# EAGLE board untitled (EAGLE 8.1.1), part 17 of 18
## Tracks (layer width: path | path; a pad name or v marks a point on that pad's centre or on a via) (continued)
S$17259 (continued)
  Bottom 0: 77.97,164.06 77.65,164.08
S$17260
  Bottom 0: 77.65,164.08 77.39,164.03
S$17261
  Bottom 0: 77.39,164.03 75.39,166.04
S$17262
  Bottom 0: 75.39,166.04 75.32,166.1
S$17263
  Bottom 0: 75.32,166.1 75.25,166.15
S$17264
  Bottom 0: 75.25,166.15 75.16,166.18
S$17265
  Bottom 0: 75.16,166.18 75.08,166.2
S$17266
  Bottom 0: 75.08,166.2 74.99,166.21
S$17267
  Bottom 0: 74.99,166.21 68.93,166.21
S$17268
  Bottom 0: 68.93,166.21 68.75,166.33
S$17269
  Bottom 0: 68.75,166.33 68.45,166.44
S$17270
  Bottom 0: 68.45,166.44 68.12,166.46
S$17271
  Bottom 0: 68.12,166.46 67.8,166.4
S$17272
  Bottom 0: 67.8,166.4 67.79,166.38
S$17273
  Bottom 0: 67.79,166.38 80.91,179.51
S$17274
  Bottom 0: 80.91,179.51 81.03,179.51
S$17275
  Bottom 0: 81.03,179.51 81.03,177.8
S$17276
  Bottom 0: 81.03,177.8 81.04,177.72
S$17277
  Bottom 0: 81.04,177.72 81.08,177.65
S$17278
  Bottom 0: 81.08,177.65 81.14,177.6
S$17279
  Bottom 0: 81.14,177.6 81.21,177.56
S$17280
  Bottom 0: 81.21,177.56 81.28,177.55
S$17281
  Bottom 0: 81.28,177.55 81.67,177.55
S$17282
  Bottom 0: 81.67,177.55 79.01,174.88
S$17283
  Bottom 0: 79.01,174.88 78.97,174.83
S$17284
  Bottom 0: 78.97,174.83 78.93,174.77
S$17285
  Bottom 0: 78.93,174.77 78.9,174.71
S$17286
  Bottom 0: 78.9,174.71 78.89,174.64
S$17287
  Bottom 0: 78.89,174.64 78.88,174.57
S$17288
  Bottom 0: 78.88,174.57 78.88,166.19
S$17289
  Bottom 0: 78.88,166.19 78.71,166.03
S$17290
  Bottom 0: 78.71,166.03 78.54,165.75
S$17291
  Bottom 0: 78.54,165.75 78.46,165.43
S$17292
  Bottom 0: 78.46,165.43 78.46,165.11
S$17293
  Bottom 0: 78.46,165.11 78.54,164.79
S$17294
  Bottom 0: 78.54,164.79 78.71,164.52
S$17295
  Bottom 0: 78.71,164.52 78.95,164.3
S$17296
  Bottom 0: 78.95,164.3 79.24,164.15
S$17297
  Bottom 0: 79.24,164.15 79.56,164.08
S$17298
  Bottom 0: 79.56,164.08 79.88,164.1
S$17299
  Bottom 0: 79.88,164.1 80.19,164.21
S$17300
  Bottom 0: 80.19,164.21 80.45,164.4
S$17301
  Bottom 0: 80.45,164.4 80.66,164.65
S$17302
  Bottom 0: 80.66,164.65 80.78,164.95
S$17303
  Bottom 0: 80.78,164.95 80.83,165.27
S$17304
  Bottom 0: 80.83,165.27 80.78,165.59
S$17305
  Bottom 0: 80.78,165.59 80.66,165.89
S$17306
  Bottom 0: 80.66,165.89 80.45,166.15
S$17307
  Bottom 0: 80.45,166.15 80.19,166.33
S$17308
  Bottom 0: 80.19,166.33 79.88,166.44
S$17309
  Bottom 0: 79.88,166.44 79.76,166.44
S$17310
  Bottom 0: 79.76,166.44 79.76,167.73
S$17311
  Bottom 0: 79.76,167.73 79.78,167.71
S$17312
  Bottom 0: 79.78,167.71 80.02,167.45
S$17313
  Bottom 0: 80.02,167.45 80.31,167.26
S$17314
  Bottom 0: 80.31,167.26 80.64,167.16
S$17315
  Bottom 0: 80.64,167.16 80.99,167.14
S$17316
  Bottom 0: 80.99,167.14 81.34,167.2
S$17317
  Bottom 0: 81.34,167.2 81.65,167.35
S$17318
  Bottom 0: 81.65,167.35 81.92,167.57
S$17319
  Bottom 0: 81.92,167.57 82.13,167.86
S$17320
  Bottom 0: 82.13,167.86 82.25,168.18
S$17321
  Bottom 0: 82.25,168.18 82.3,168.53
S$17322
  Bottom 0: 82.3,168.53 82.25,168.87
S$17323
  Bottom 0: 82.25,168.87 82.13,169.2
S$17324
  Bottom 0: 82.13,169.2 81.92,169.48
S$17325
  Bottom 0: 81.92,169.48 81.65,169.71
S$17326
  Bottom 0: 81.65,169.71 81.34,169.86
S$17327
  Bottom 0: 81.34,169.86 80.99,169.92
S$17328
  Bottom 0: 80.99,169.92 80.64,169.9
S$17329
  Bottom 0: 80.64,169.9 80.31,169.79
S$17330
  Bottom 0: 80.31,169.79 80.02,169.61
S$17331
  Bottom 0: 80.02,169.61 79.78,169.35
S$17332
  Bottom 0: 79.78,169.35 79.76,169.34
S$17333
  Bottom 0: 79.76,169.34 79.76,174.38
S$17334
  Bottom 0: 79.76,174.38 82.49,177.1
S$17335
  Bottom 0: 82.49,177.1 82.53,177.17
S$17336
  Bottom 0: 82.53,177.17 82.56,177.2
S$17337
  Bottom 0: 82.56,177.2 82.56,177.24
S$17338
  Bottom 0: 82.56,177.24 82.6,177.3
S$17339
  Bottom 0: 82.6,177.3 82.6,177.36
S$17340
  Bottom 0: 82.6,177.36 82.62,177.42
S$17341
  Bottom 0: 82.62,177.42 82.62,177.55
S$17342
  Bottom 0: 82.62,177.55 83.06,177.55
S$17343
  Bottom 0: 83.06,177.55 83.14,177.56
S$17344
  Bottom 0: 83.14,177.56 83.21,177.6
S$17345
  Bottom 0: 83.21,177.6 83.27,177.65
S$17346
  Bottom 0: 83.27,177.65 83.31,177.72
S$17347
  Bottom 0: 83.31,177.72 83.32,177.8
S$17348
  Bottom 0: 83.32,177.8 83.32,179.51
S$17349
  Bottom 0: 83.32,179.51 83.92,179.51
S$17350
  Bottom 0: 83.92,179.51 83.75,179.31
S$17351
  Bottom 0: 83.75,179.31 83.62,179.01
S$17352
  Bottom 0: 83.62,179.01 83.57,178.69
S$17353
  Bottom 0: 83.57,178.69 83.62,178.37
S$17354
  Bottom 0: 83.62,178.37 83.75,178.07
S$17355
  Bottom 0: 83.75,178.07 83.97,177.82
S$17356
  Bottom 0: 83.97,177.82 84.24,177.65
S$17357
  Bottom 0: 84.24,177.65 84.55,177.56
S$17358
  Bottom 0: 84.55,177.56 84.88,177.56
S$17359
  Bottom 0: 84.88,177.56 85.19,177.65
S$17360
  Bottom 0: 85.19,177.65 85.46,177.82
S$17361
  Bottom 0: 85.46,177.82 85.67,178.07
S$17362
  Bottom 0: 85.67,178.07 85.81,178.37
S$17363
  Bottom 0: 85.81,178.37 85.86,178.69
S$17364
  Bottom 0: 85.86,178.69 85.81,179.01
S$17365
  Bottom 0: 85.81,179.01 85.67,179.31
S$17366
  Bottom 0: 85.67,179.31 85.5,179.51
S$17367
  Bottom 0: 85.5,179.51 100.08,179.51
S$17368
  Bottom 0: 100.08,179.51 100.08,177.8
S$17369
  Bottom 0: 100.08,177.8 100.09,177.72
S$17370
  Bottom 0: 100.09,177.72 100.13,177.65
S$17371
  Bottom 0: 100.13,177.65 100.18,177.6
S$17372
  Bottom 0: 100.18,177.6 100.25,177.56
S$17373
  Bottom 0: 100.25,177.56 100.33,177.55
S$17374
  Bottom 0: 100.33,177.55 100.72,177.55
S$17375
  Bottom 0: 100.72,177.55 97.88,174.71
S$17376
  Bottom 0: 97.88,174.71 97.83,174.66
S$17377
  Bottom 0: 97.83,174.66 97.8,174.6
S$17378
  Bottom 0: 97.8,174.6 97.77,174.53
S$17379
  Bottom 0: 97.77,174.53 97.75,174.47
S$17380
  Bottom 0: 97.75,174.47 97.75,174.4
S$17381
  Bottom 0: 97.75,174.4 97.75,165.99
S$17382
  Bottom 0: 97.75,165.99 97.59,165.75
S$17383
  Bottom 0: 97.59,165.75 97.51,165.43
S$17384
  Bottom 0: 97.51,165.43 97.51,165.1
S$17385
  Bottom 0: 97.51,165.1 97.59,164.79
S$17386
  Bottom 0: 97.59,164.79 97.67,164.67
S$17387
  Bottom 0: 97.67,164.67 95.44,166.9
S$17388
  Bottom 0: 95.44,166.9 95.38,166.94
S$17389
  Bottom 0: 95.38,166.94 95.32,166.98
S$17390
  Bottom 0: 95.32,166.98 95.26,167
S$17391
  Bottom 0: 95.26,167 95.19,167.02
S$17392
  Bottom 0: 95.19,167.02 95.12,167.03
S$17393
  Bottom 0: 95.12,167.03 91.92,167.03
S$17394
  Bottom 0: 91.92,167.03 88.5,170.45
S$17395
  Bottom 0: 88.5,170.45 88.61,170.72
S$17396
  Bottom 0: 88.61,170.72 88.65,171.07
S$17397
  Bottom 0: 88.65,171.07 88.61,171.41
S$17398
  Bottom 0: 88.61,171.41 88.48,171.74
S$17399
  Bottom 0: 88.48,171.74 88.27,172.02
S$17400
  Bottom 0: 88.27,172.02 88,172.25
S$17401
  Bottom 0: 88,172.25 87.69,172.4
S$17402
  Bottom 0: 87.69,172.4 87.34,172.46
S$17403
  Bottom 0: 87.34,172.46 86.99,172.44
S$17404
  Bottom 0: 86.99,172.44 86.66,172.33
S$17405
  Bottom 0: 86.66,172.33 86.36,172.15
S$17406
  Bottom 0: 86.36,172.15 86.13,171.89
S$17407
  Bottom 0: 86.13,171.89 85.95,171.58
S$17408
  Bottom 0: 85.95,171.58 85.86,171.24
S$17409
  Bottom 0: 85.86,171.24 85.86,170.9
S$17410
  Bottom 0: 85.86,170.9 85.95,170.56
S$17411
  Bottom 0: 85.95,170.56 86.13,170.25
S$17412
  Bottom 0: 86.13,170.25 86.36,169.99
S$17413
  Bottom 0: 86.36,169.99 86.66,169.8
S$17414
  Bottom 0: 86.66,169.8 86.99,169.7
S$17415
  Bottom 0: 86.99,169.7 87.34,169.68
S$17416
  Bottom 0: 87.34,169.68 87.69,169.74
S$17417
  Bottom 0: 87.69,169.74 87.87,169.83
S$17418
  Bottom 0: 87.87,169.83 91.42,166.27
S$17419
  Bottom 0: 91.42,166.27 91.48,166.23
S$17420
  Bottom 0: 91.48,166.23 91.53,166.19
S$17421
  Bottom 0: 91.53,166.19 91.6,166.16
S$17422
  Bottom 0: 91.6,166.16 91.66,166.15
S$17423
  Bottom 0: 91.66,166.15 91.73,166.14
S$17424
  Bottom 0: 91.73,166.14 94.94,166.14
S$17425
  Bottom 0: 94.94,166.14 97.01,164.06
S$17426
  Bottom 0: 97.01,164.06 96.7,164.08
S$17427
  Bottom 0: 96.7,164.08 96.45,164.03
S$17428
  Bottom 0: 96.45,164.03 94.81,165.67
S$17429
  Bottom 0: 94.81,165.67 94.74,165.74
S$17430
  Bottom 0: 94.74,165.74 94.67,165.78
S$17431
  Bottom 0: 94.67,165.78 94.58,165.81
S$17432
  Bottom 0: 94.58,165.81 94.5,165.84
S$17433
  Bottom 0: 94.5,165.84 94.4,165.84
S$17434
  Bottom 0: 94.4,165.84 88.3,165.84
S$17435
  Bottom 0: 88.3,165.84 88.28,165.89
S$17436
  Bottom 0: 88.28,165.89 88.07,166.15
S$17437
  Bottom 0: 88.07,166.15 87.81,166.33
S$17438
  Bottom 0: 87.81,166.33 87.5,166.44
S$17439
  Bottom 0: 87.5,166.44 87.18,166.46
S$17440
  Bottom 0: 87.18,166.46 86.86,166.4
S$17441
  Bottom 0: 86.86,166.4 86.57,166.25
S$17442
  Bottom 0: 86.57,166.25 86.33,166.03
S$17443
  Bottom 0: 86.33,166.03 86.16,165.75
S$17444
  Bottom 0: 86.16,165.75 86.08,165.43
S$17445
  Bottom 0: 86.08,165.43 86.08,165.11
S$17446
  Bottom 0: 86.08,165.11 86.12,164.94
S$17447
  Bottom 0: 86.12,164.94 84.65,163.46
S$17448
  Bottom 0: 84.65,163.46 78.77,163.46
S$17449
  Bottom 0: 93.05,169.02 93.34,169.09
S$17450
  Bottom 0: 93.34,169.09 93.61,169.24
S$17451
  Bottom 0: 93.61,169.24 93.81,169.46
S$17452
  Bottom 0: 93.81,169.46 93.94,169.73
S$17453
  Bottom 0: 93.94,169.73 93.99,170.03
S$17454
  Bottom 0: 93.99,170.03 93.94,170.33
S$17455
  Bottom 0: 93.94,170.33 93.81,170.61
S$17456
  Bottom 0: 93.81,170.61 93.61,170.82
S$17457
  Bottom 0: 93.61,170.82 93.34,170.98
S$17458
  Bottom 0: 93.34,170.98 93.05,171.04
S$17459
  Bottom 0: 93.05,171.04 92.75,171.02
S$17460
  Bottom 0: 92.75,171.02 92.47,170.91
S$17461
  Bottom 0: 92.47,170.91 92.23,170.72
S$17462
  Bottom 0: 92.23,170.72 92.06,170.47
S$17463
  Bottom 0: 92.06,170.47 91.97,170.19
S$17464
  Bottom 0: 91.97,170.19 91.97,169.88
S$17465
  Bottom 0: 91.97,169.88 92.06,169.59
S$17466
  Bottom 0: 92.06,169.59 92.23,169.34
S$17467
  Bottom 0: 92.23,169.34 92.47,169.15
S$17468
  Bottom 0: 92.47,169.15 92.75,169.04
S$17469
  Bottom 0: 92.75,169.04 93.05,169.02
S$17470
  Bottom 0: 75.19,169.03 75.48,169.09
S$17471
  Bottom 0: 75.48,169.09 75.75,169.25
S$17472
  Bottom 0: 75.75,169.25 75.95,169.46
S$17473
  Bottom 0: 75.95,169.46 76.08,169.74
S$17474
  Bottom 0: 76.08,169.74 76.13,170.04
S$17475
  Bottom 0: 76.13,170.04 76.08,170.34
S$17476
  Bottom 0: 76.08,170.34 75.95,170.61
S$17477
  Bottom 0: 75.95,170.61 75.75,170.83
S$17478
  Bottom 0: 75.75,170.83 75.48,170.98
S$17479
  Bottom 0: 75.48,170.98 75.19,171.05
S$17480
  Bottom 0: 75.19,171.05 74.88,171.03
S$17481
  Bottom 0: 74.88,171.03 74.61,170.92
S$17482
  Bottom 0: 74.61,170.92 74.36,170.73
S$17483
  Bottom 0: 74.36,170.73 74.2,170.48
S$17484
  Bottom 0: 74.2,170.48 74.11,170.19
S$17485
  Bottom 0: 74.11,170.19 74.11,169.88
S$17486
  Bottom 0: 74.11,169.88 74.2,169.6
S$17487
  Bottom 0: 74.2,169.6 74.36,169.35
S$17488
  Bottom 0: 74.36,169.35 74.61,169.16
S$17489
  Bottom 0: 74.61,169.16 74.88,169.05
S$17490
  Bottom 0: 74.88,169.05 75.19,169.03
S$17491
  Bottom 0: 83.44,171.32 83.89,171.37
S$17492
  Bottom 0: 83.89,171.37 84.32,171.5
S$17493
  Bottom 0: 84.32,171.5 84.71,171.71
S$17494
  Bottom 0: 84.71,171.71 85.06,171.99
S$17495
  Bottom 0: 85.06,171.99 85.34,172.34
S$17496
  Bottom 0: 85.34,172.34 85.56,172.74
S$17497
  Bottom 0: 85.56,172.74 85.68,173.16
S$17498
  Bottom 0: 85.68,173.16 85.73,173.61
S$17499
  Bottom 0: 85.73,173.61 85.68,174.06
S$17500
  Bottom 0: 85.68,174.06 85.56,174.48
S$17501
  Bottom 0: 85.56,174.48 85.34,174.88
S$17502
  Bottom 0: 85.34,174.88 85.06,175.22
S$17503
  Bottom 0: 85.06,175.22 84.71,175.51
S$17504
  Bottom 0: 84.71,175.51 84.32,175.72
S$17505
  Bottom 0: 84.32,175.72 83.89,175.85
S$17506
  Bottom 0: 83.89,175.85 83.44,175.9
S$17507
  Bottom 0: 83.44,175.9 83,175.85
S$17508
  Bottom 0: 83,175.85 82.57,175.72
S$17509
  Bottom 0: 82.57,175.72 82.17,175.51
S$17510
  Bottom 0: 82.17,175.51 81.83,175.22
S$17511
  Bottom 0: 81.83,175.22 81.54,174.88
S$17512
  Bottom 0: 81.54,174.88 81.33,174.48
S$17513
  Bottom 0: 81.33,174.48 81.2,174.06
S$17514
  Bottom 0: 81.2,174.06 81.16,173.61
S$17515
  Bottom 0: 81.16,173.61 81.2,173.16
S$17516
  Bottom 0: 81.2,173.16 81.33,172.74
S$17517
  Bottom 0: 81.33,172.74 81.54,172.34
S$17518
  Bottom 0: 81.54,172.34 81.83,171.99
S$17519
  Bottom 0: 81.83,171.99 82.17,171.71
S$17520
  Bottom 0: 82.17,171.71 82.57,171.5
S$17521
  Bottom 0: 82.57,171.5 83,171.37
S$17522
  Bottom 0: 83,171.37 83.44,171.32
S$17523
  Bottom 0: 93.05,176.64 93.34,176.71
S$17524
  Bottom 0: 93.34,176.71 93.61,176.86
S$17525
  Bottom 0: 93.61,176.86 93.81,177.08
S$17526
  Bottom 0: 93.81,177.08 93.94,177.35
S$17527
  Bottom 0: 93.94,177.35 93.99,177.65
S$17528
  Bottom 0: 93.99,177.65 93.94,177.95
S$17529
  Bottom 0: 93.94,177.95 93.81,178.23
S$17530
  Bottom 0: 93.81,178.23 93.61,178.44
S$17531
  Bottom 0: 93.61,178.44 93.34,178.6
S$17532
  Bottom 0: 93.34,178.6 93.05,178.66
S$17533
  Bottom 0: 93.05,178.66 92.75,178.64
S$17534
  Bottom 0: 92.75,178.64 92.47,178.53
S$17535
  Bottom 0: 92.47,178.53 92.23,178.34
S$17536
  Bottom 0: 92.23,178.34 92.06,178.09
S$17537
  Bottom 0: 92.06,178.09 91.97,177.81
S$17538
  Bottom 0: 91.97,177.81 91.97,177.5
S$17539
  Bottom 0: 91.97,177.5 92.06,177.21
S$17540
  Bottom 0: 92.06,177.21 92.23,176.96
S$17541
  Bottom 0: 92.23,176.96 92.47,176.77
S$17542
  Bottom 0: 92.47,176.77 92.75,176.66
S$17543
  Bottom 0: 92.75,176.66 93.05,176.64
S$17544
  Bottom 0: 137.44,164.28 137.61,164.39
S$17545
  Bottom 0: 137.61,164.39 137.81,164.65
S$17546
  Bottom 0: 137.81,164.65 137.94,164.95
S$17547
  Bottom 0: 137.94,164.95 137.99,165.27
S$17548
  Bottom 0: 137.99,165.27 137.94,165.59
S$17549
  Bottom 0: 137.94,165.59 137.81,165.89
S$17550
  Bottom 0: 137.81,165.89 137.61,166.14
S$17551
  Bottom 0: 137.61,166.14 137.34,166.33
S$17552
  Bottom 0: 137.34,166.33 137.04,166.44
S$17553
  Bottom 0: 137.04,166.44 136.8,166.45
S$17554
  Bottom 0: 136.8,166.45 136.8,167.91
S$17555
  Bottom 0: 136.8,167.91 136.92,167.71
S$17556
  Bottom 0: 136.92,167.71 137.16,167.45
S$17557
  Bottom 0: 137.16,167.45 137.46,167.26
S$17558
  Bottom 0: 137.46,167.26 137.78,167.16
S$17559
  Bottom 0: 137.78,167.16 138.13,167.14
S$17560
  Bottom 0: 138.13,167.14 138.48,167.2
S$17561
  Bottom 0: 138.48,167.2 138.8,167.35
S$17562
  Bottom 0: 138.8,167.35 139.06,167.57
S$17563
  Bottom 0: 139.06,167.57 139.27,167.86
S$17564
  Bottom 0: 139.27,167.86 139.4,168.18
S$17565
  Bottom 0: 139.4,168.18 139.45,168.53
S$17566
  Bottom 0: 139.45,168.53 139.4,168.87
S$17567
  Bottom 0: 139.4,168.87 139.29,169.15
S$17568
  Bottom 0: 139.29,169.15 142.17,166.27
S$17569
  Bottom 0: 142.17,166.27 142.22,166.22
S$17570
  Bottom 0: 142.22,166.22 142.28,166.18
S$17571
  Bottom 0: 142.28,166.18 142.34,166.16
S$17572
  Bottom 0: 142.34,166.16 142.41,166.14
S$17573
  Bottom 0: 142.41,166.14 142.48,166.14
S$17574
  Bottom 0: 142.48,166.14 143.61,166.14
S$17575
  Bottom 0: 143.61,166.14 143.49,166.02
S$17576
  Bottom 0: 143.49,166.02 143.32,165.75
S$17577
  Bottom 0: 143.32,165.75 143.23,165.43
S$17578
  Bottom 0: 143.23,165.43 143.23,165.1
S$17579
  Bottom 0: 143.23,165.1 143.32,164.79
S$17580
  Bottom 0: 143.32,164.79 143.49,164.52
S$17581
  Bottom 0: 143.49,164.52 143.72,164.29
S$17582
  Bottom 0: 143.72,164.29 143.75,164.28
S$17583
  Bottom 0: 143.75,164.28 137.44,164.28
S$17584
  Bottom 0: 118.55,164.4 118.76,164.65
S$17585
  Bottom 0: 118.76,164.65 118.89,164.95
S$17586
  Bottom 0: 118.89,164.95 118.93,165.27
S$17587
  Bottom 0: 118.93,165.27 118.89,165.59
S$17588
  Bottom 0: 118.89,165.59 118.76,165.89
S$17589
  Bottom 0: 118.76,165.89 118.55,166.15
S$17590
  Bottom 0: 118.55,166.15 118.29,166.33
S$17591
  Bottom 0: 118.29,166.33 117.98,166.44
S$17592
  Bottom 0: 117.98,166.44 117.87,166.44
S$17593
  Bottom 0: 117.87,166.44 117.87,167.72
S$17594
  Bottom 0: 117.87,167.72 117.87,167.71
S$17595
  Bottom 0: 117.87,167.71 118.11,167.45
S$17596
  Bottom 0: 118.11,167.45 118.41,167.26
S$17597
  Bottom 0: 118.41,167.26 118.73,167.16
S$17598
  Bottom 0: 118.73,167.16 119.08,167.14
S$17599
  Bottom 0: 119.08,167.14 119.43,167.2
S$17600
  Bottom 0: 119.43,167.2 119.75,167.35
S$17601
  Bottom 0: 119.75,167.35 120.02,167.57
S$17602
  Bottom 0: 120.02,167.57 120.22,167.86
S$17603
  Bottom 0: 120.22,167.86 120.35,168.18
S$17604
  Bottom 0: 120.35,168.18 120.4,168.53
S$17605
  Bottom 0: 120.4,168.53 120.35,168.87
S$17606
  Bottom 0: 120.35,168.87 120.22,169.2
S$17607
  Bottom 0: 120.22,169.2 120.02,169.48
S$17608
  Bottom 0: 120.02,169.48 119.75,169.71
S$17609
  Bottom 0: 119.75,169.71 119.43,169.86
S$17610
  Bottom 0: 119.43,169.86 119.08,169.92
S$17611
  Bottom 0: 119.08,169.92 118.73,169.9
S$17612
  Bottom 0: 118.73,169.9 118.41,169.79
S$17613
  Bottom 0: 118.41,169.79 118.11,169.61
S$17614
  Bottom 0: 118.11,169.61 117.87,169.35
S$17615
  Bottom 0: 117.87,169.35
S$17616
  Bottom 0: 117.87,169.35 117.87,174.4
S$17617
  Bottom 0: 117.87,174.4 120.58,177.1
S$17618
  Bottom 0: 120.58,177.1 120.61,177.16
S$17619
  Bottom 0: 120.61,177.16 120.65,177.2
S$17620
  Bottom 0: 120.65,177.2 120.66,177.25
S$17621
  Bottom 0: 120.66,177.25 120.69,177.3
S$17622
  Bottom 0: 120.69,177.3 120.69,177.36
S$17623
  Bottom 0: 120.69,177.36 120.71,177.42
S$17624
  Bottom 0: 120.71,177.42 120.71,177.55
S$17625
  Bottom 0: 120.71,177.55 121.16,177.55
S$17626
  Bottom 0: 121.16,177.55 121.23,177.56
S$17627
  Bottom 0: 121.23,177.56 121.31,177.6
S$17628
  Bottom 0: 121.31,177.6 121.36,177.65
S$17629
  Bottom 0: 121.36,177.65 121.4,177.72
S$17630
  Bottom 0: 121.4,177.72 121.41,177.8
S$17631
  Bottom 0: 121.41,177.8 121.41,179.51
S$17632
  Bottom 0: 121.41,179.51 122.02,179.51
S$17633
  Bottom 0: 122.02,179.51 121.85,179.31
S$17634
  Bottom 0: 121.85,179.31 121.71,179.01
S$17635
  Bottom 0: 121.71,179.01 121.67,178.69
S$17636
  Bottom 0: 121.67,178.69 121.71,178.37
S$17637
  Bottom 0: 121.71,178.37 121.85,178.07
S$17638
  Bottom 0: 121.85,178.07 122.06,177.82
S$17639
  Bottom 0: 122.06,177.82 122.34,177.65
S$17640
  Bottom 0: 122.34,177.65 122.65,177.56
S$17641
  Bottom 0: 122.65,177.56 122.97,177.56
S$17642
  Bottom 0: 122.97,177.56 123.28,177.65
S$17643
  Bottom 0: 123.28,177.65 123.56,177.82
S$17644
  Bottom 0: 123.56,177.82 123.77,178.07
S$17645
  Bottom 0: 123.77,178.07 123.91,178.37
S$17646
  Bottom 0: 123.91,178.37 123.95,178.69
S$17647
  Bottom 0: 123.95,178.69 123.91,179.01
S$17648
  Bottom 0: 123.91,179.01 123.77,179.31
S$17649
  Bottom 0: 123.77,179.31 123.6,179.51
S$17650
  Bottom 0: 123.6,179.51 138.18,179.51
S$17651
  Bottom 0: 138.18,179.51 138.18,177.8
S$17652
  Bottom 0: 138.18,177.8 138.19,177.72
S$17653
  Bottom 0: 138.19,177.72 138.23,177.65
S$17654
  Bottom 0: 138.23,177.65 138.28,177.6
S$17655
  Bottom 0: 138.28,177.6 138.35,177.56
S$17656
  Bottom 0: 138.35,177.56 138.43,177.55
S$17657
  Bottom 0: 138.43,177.55 138.82,177.55
S$17658
  Bottom 0: 138.82,177.55 136.05,174.78
S$17659
  Bottom 0: 136.05,174.78 136.01,174.73
S$17660
  Bottom 0: 136.01,174.73 135.97,174.67
S$17661
  Bottom 0: 135.97,174.67 135.94,174.6
S$17662
  Bottom 0: 135.94,174.6 135.93,174.54
S$17663
  Bottom 0: 135.93,174.54 135.92,174.47
S$17664
  Bottom 0: 135.92,174.47 135.92,166.07
S$17665
  Bottom 0: 135.92,166.07 135.87,166.02
S$17666
  Bottom 0: 135.87,166.02 135.7,165.75
S$17667
  Bottom 0: 135.7,165.75 135.61,165.43
S$17668
  Bottom 0: 135.61,165.43 135.61,165.1
S$17669
  Bottom 0: 135.61,165.1 135.7,164.79
S$17670
  Bottom 0: 135.7,164.79 135.79,164.64
S$17671
  Bottom 0: 135.79,164.64 133.54,166.89
S$17672
  Bottom 0: 133.54,166.89 133.49,166.94
S$17673
  Bottom 0: 133.49,166.94 133.43,166.97
S$17674
  Bottom 0: 133.43,166.97 133.36,167
S$17675
  Bottom 0: 133.36,167 133.3,167.02
S$17676
  Bottom 0: 133.3,167.02 133.23,167.03
S$17677
  Bottom 0: 133.23,167.03 122.76,167.03
S$17678
  Bottom 0: 122.76,167.03 122.69,167.02
S$17679
  Bottom 0: 122.69,167.02 122.63,167
S$17680
  Bottom 0: 122.63,167 122.56,166.98
S$17681
  Bottom 0: 122.56,166.98 122.5,166.94
S$17682
  Bottom 0: 122.5,166.94 122.45,166.9
S$17683
  Bottom 0: 122.45,166.9 119.95,164.4
S$17684
  Bottom 0: 119.95,164.4 118.55,164.4
S$17685
  Bottom 0: 131.16,169.02 131.45,169.09
S$17686
  Bottom 0: 131.45,169.09 131.71,169.24
S$17687
  Bottom 0: 131.71,169.24 131.92,169.46
S$17688
  Bottom 0: 131.92,169.46 132.05,169.73
S$17689
  Bottom 0: 132.05,169.73 132.09,170.03
S$17690
  Bottom 0: 132.09,170.03 132.05,170.33
S$17691
  Bottom 0: 132.05,170.33 131.92,170.61
S$17692
  Bottom 0: 131.92,170.61 131.71,170.82
S$17693
  Bottom 0: 131.71,170.82 131.45,170.98
S$17694
  Bottom 0: 131.45,170.98 131.16,171.04
S$17695
  Bottom 0: 131.16,171.04 130.85,171.02
S$17696
  Bottom 0: 130.85,171.02 130.57,170.91
S$17697
  Bottom 0: 130.57,170.91 130.33,170.72
S$17698
  Bottom 0: 130.33,170.72 130.16,170.47
S$17699
  Bottom 0: 130.16,170.47 130.07,170.19
S$17700
  Bottom 0: 130.07,170.19 130.07,169.88
S$17701
  Bottom 0: 130.07,169.88 130.16,169.59
S$17702
  Bottom 0: 130.16,169.59 130.33,169.34
S$17703
  Bottom 0: 130.33,169.34 130.57,169.15
S$17704
  Bottom 0: 130.57,169.15 130.85,169.04
S$17705
  Bottom 0: 130.85,169.04 131.16,169.02
S$17706
  Bottom 0: 125.44,169.68 125.78,169.74
S$17707
  Bottom 0: 125.78,169.74 126.1,169.89
S$17708
  Bottom 0: 126.1,169.89 126.36,170.11
S$17709
  Bottom 0: 126.36,170.11 126.57,170.4
S$17710
  Bottom 0: 126.57,170.4 126.7,170.72
S$17711
  Bottom 0: 126.7,170.72 126.75,171.07
S$17712
  Bottom 0: 126.75,171.07 126.7,171.41
S$17713
  Bottom 0: 126.7,171.41 126.57,171.74
S$17714
  Bottom 0: 126.57,171.74 126.36,172.02
S$17715
  Bottom 0: 126.36,172.02 126.1,172.25
S$17716
  Bottom 0: 126.1,172.25 125.78,172.4
S$17717
  Bottom 0: 125.78,172.4 125.44,172.46
S$17718
  Bottom 0: 125.44,172.46 125.08,172.44
S$17719
  Bottom 0: 125.08,172.44 124.75,172.33
S$17720
  Bottom 0: 124.75,172.33 124.46,172.15
S$17721
  Bottom 0: 124.46,172.15 124.22,171.89
S$17722
  Bottom 0: 124.22,171.89 124.05,171.58
S$17723
  Bottom 0: 124.05,171.58 123.96,171.24
S$17724
  Bottom 0: 123.96,171.24 123.96,170.9
S$17725
  Bottom 0: 123.96,170.9 124.05,170.56
S$17726
  Bottom 0: 124.05,170.56 124.22,170.25
S$17727
  Bottom 0: 124.22,170.25 124.46,169.99
S$17728
  Bottom 0: 124.46,169.99 124.75,169.8
S$17729
  Bottom 0: 124.75,169.8 125.08,169.7
S$17730
  Bottom 0: 125.08,169.7 125.44,169.68
S$17731
  Bottom 0: 121.54,171.32 121.99,171.37
S$17732
  Bottom 0: 121.99,171.37 122.41,171.5
S$17733
  Bottom 0: 122.41,171.5 122.81,171.71
S$17734
  Bottom 0: 122.81,171.71 123.15,171.99
S$17735
  Bottom 0: 123.15,171.99 123.44,172.34
S$17736
  Bottom 0: 123.44,172.34 123.65,172.74
S$17737
  Bottom 0: 123.65,172.74 123.78,173.16
S$17738
  Bottom 0: 123.78,173.16 123.83,173.61
S$17739
  Bottom 0: 123.83,173.61 123.78,174.06
S$17740
  Bottom 0: 123.78,174.06 123.65,174.48
S$17741
  Bottom 0: 123.65,174.48 123.44,174.88
S$17742
  Bottom 0: 123.44,174.88 123.15,175.22
S$17743
  Bottom 0: 123.15,175.22 122.81,175.51
S$17744
  Bottom 0: 122.81,175.51 122.41,175.72
S$17745
  Bottom 0: 122.41,175.72 121.99,175.85
S$17746
  Bottom 0: 121.99,175.85 121.54,175.9
S$17747
  Bottom 0: 121.54,175.9 121.09,175.85
S$17748
  Bottom 0: 121.09,175.85 120.66,175.72
S$17749
  Bottom 0: 120.66,175.72 120.27,175.51
S$17750
  Bottom 0: 120.27,175.51 119.92,175.22
S$17751
  Bottom 0: 119.92,175.22 119.64,174.88
S$17752
  Bottom 0: 119.64,174.88 119.42,174.48
S$17753
  Bottom 0: 119.42,174.48 119.3,174.06
S$17754
  Bottom 0: 119.3,174.06 119.25,173.61
S$17755
  Bottom 0: 119.25,173.61 119.3,173.16
S$17756
  Bottom 0: 119.3,173.16 119.42,172.74
S$17757
  Bottom 0: 119.42,172.74 119.64,172.34
S$17758
  Bottom 0: 119.64,172.34 119.92,171.99
S$17759
  Bottom 0: 119.92,171.99 120.27,171.71
S$17760
  Bottom 0: 120.27,171.71 120.66,171.5
S$17761
  Bottom 0: 120.66,171.5 121.09,171.37
S$17762
  Bottom 0: 121.09,171.37 121.54,171.32
S$17763
  Bottom 0: 131.16,176.64 131.45,176.71
S$17764
  Bottom 0: 131.45,176.71 131.71,176.86
S$17765
  Bottom 0: 131.71,176.86 131.92,177.08
S$17766
  Bottom 0: 131.92,177.08 132.05,177.35
S$17767
  Bottom 0: 132.05,177.35 132.09,177.65
S$17768
  Bottom 0: 132.09,177.65 132.05,177.95
S$17769
  Bottom 0: 132.05,177.95 131.92,178.23
S$17770
  Bottom 0: 131.92,178.23 131.71,178.44
S$17771
  Bottom 0: 131.71,178.44 131.45,178.6
S$17772
  Bottom 0: 131.45,178.6 131.16,178.66
S$17773
  Bottom 0: 131.16,178.66 130.85,178.64
S$17774
  Bottom 0: 130.85,178.64 130.57,178.53
S$17775
  Bottom 0: 130.57,178.53 130.33,178.34
S$17776
  Bottom 0: 130.33,178.34 130.16,178.09
S$17777
  Bottom 0: 130.16,178.09 130.07,177.81
S$17778
  Bottom 0: 130.07,177.81 130.07,177.5
S$17779
  Bottom 0: 130.07,177.5 130.16,177.21
S$17780
  Bottom 0: 130.16,177.21 130.33,176.96
S$17781
  Bottom 0: 130.33,176.96 130.57,176.77
S$17782
  Bottom 0: 130.57,176.77 130.85,176.66
S$17783
  Bottom 0: 130.85,176.66 131.16,176.64
S$17784
  Bottom 0: 173.72,165.2 171.83,167.09
S$17785
  Bottom 0: 171.83,167.09 171.78,167.13
S$17786
  Bottom 0: 171.78,167.13 171.71,167.17
S$17787
  Bottom 0: 171.71,167.17 171.65,167.19
S$17788
  Bottom 0: 171.65,167.19 171.59,167.21
S$17789
  Bottom 0: 171.59,167.21 171.52,167.21
S$17790
  Bottom 0: 171.52,167.21 167.94,167.21
S$17791
  Bottom 0: 167.94,167.21 164.69,170.45
S$17792
  Bottom 0: 164.69,170.45 164.8,170.72
S$17793
  Bottom 0: 164.8,170.72 164.85,171.07
S$17794
  Bottom 0: 164.85,171.07 164.8,171.41
S$17795
  Bottom 0: 164.8,171.41 164.67,171.74
S$17796
  Bottom 0: 164.67,171.74 164.47,172.02
S$17797
  Bottom 0: 164.47,172.02 164.2,172.25
S$17798
  Bottom 0: 164.2,172.25 163.88,172.4
S$17799
  Bottom 0: 163.88,172.4 163.53,172.46
S$17800
  Bottom 0: 163.53,172.46 163.19,172.44
S$17801
  Bottom 0: 163.19,172.44 162.85,172.33
S$17802
  Bottom 0: 162.85,172.33 162.56,172.15
S$17803
  Bottom 0: 162.56,172.15 162.32,171.89
S$17804
  Bottom 0: 162.32,171.89 162.25,171.75
S$17805
  Bottom 0: 162.25,171.75 162.25,171.84
S$17806
  Bottom 0: 162.25,171.84 162.56,172.16
S$17807
  Bottom 0: 162.56,172.16 162.63,172.23
S$17808
  Bottom 0: 162.63,172.23 162.67,172.3
S$17809
  Bottom 0: 162.67,172.3 162.71,172.38
S$17810
  Bottom 0: 162.71,172.38 162.73,172.47
S$17811
  Bottom 0: 162.73,172.47 162.73,172.56
S$17812
  Bottom 0: 162.73,172.56 162.73,177.43
S$17813
  Bottom 0: 162.73,177.43 162.73,177.53
S$17814
  Bottom 0: 162.73,177.53 162.71,177.61
S$17815
  Bottom 0: 162.71,177.61 162.67,177.69
S$17816
  Bottom 0: 162.67,177.69 162.63,177.77
S$17817
  Bottom 0: 162.63,177.77 162.56,177.84
S$17818
  Bottom 0: 162.56,177.84 162.01,178.39
S$17819
  Bottom 0: 162.01,178.39 162.05,178.69
S$17820
  Bottom 0: 162.05,178.69 162.01,179.01
S$17821
  Bottom 0: 162.01,179.01 161.87,179.31
S$17822
  Bottom 0: 161.87,179.31 161.7,179.51
S$17823
  Bottom 0: 161.7,179.51 176.28,179.51
S$17824
  Bottom 0: 176.28,179.51 176.28,177.8
S$17825
  Bottom 0: 176.28,177.8 176.29,177.72
S$17826
  Bottom 0: 176.29,177.72 176.33,177.65
S$17827
  Bottom 0: 176.33,177.65 176.38,177.6
S$17828
  Bottom 0: 176.38,177.6 176.45,177.56
S$17829
  Bottom 0: 176.45,177.56 176.53,177.55
S$17830
  Bottom 0: 176.53,177.55 176.92,177.55
S$17831
  Bottom 0: 176.92,177.55 174.31,174.94
S$17832
  Bottom 0: 174.31,174.94 174.26,174.88
S$17833
  Bottom 0: 174.26,174.88 174.22,174.82
S$17834
  Bottom 0: 174.22,174.82 174.19,174.76
S$17835
  Bottom 0: 174.19,174.76 174.18,174.69
S$17836
  Bottom 0: 174.18,174.69 174.17,174.62
S$17837
  Bottom 0: 174.17,174.62 174.17,166.21
S$17838
  Bottom 0: 174.17,166.21 173.97,166.02
S$17839
  Bottom 0: 173.97,166.02 173.8,165.75
S$17840
  Bottom 0: 173.8,165.75 173.72,165.43
S$17841
  Bottom 0: 173.72,165.43 173.72,165.2
S$17842
  Bottom 0: 168.93,168.1 169.44,168.1
S$17843
  Bottom 0: 169.44,168.1 169.95,168.19
S$17844
  Bottom 0: 169.95,168.19 170.44,168.36
S$17845
  Bottom 0: 170.44,168.36 170.9,168.6
S$17846
  Bottom 0: 170.9,168.6 171.31,168.92
S$17847
  Bottom 0: 171.31,168.92 171.66,169.3
S$17848
  Bottom 0: 171.66,169.3 171.94,169.73
S$17849
  Bottom 0: 171.94,169.73 172.15,170.21
S$17850
  Bottom 0: 172.15,170.21 172.28,170.71
S$17851
  Bottom 0: 172.28,170.71 172.32,171.23
S$17852
  Bottom 0: 172.32,171.23 172.28,171.75
S$17853
  Bottom 0: 172.28,171.75 172.15,172.24
S$17854
  Bottom 0: 172.15,172.24 171.94,172.72
S$17855
  Bottom 0: 171.94,172.72 171.66,173.15
S$17856
  Bottom 0: 171.66,173.15 171.31,173.53
S$17857
  Bottom 0: 171.31,173.53 170.9,173.85
S$17858
  Bottom 0: 170.9,173.85 170.44,174.1
S$17859
  Bottom 0: 170.44,174.1 169.95,174.26
S$17860
  Bottom 0: 169.95,174.26 169.44,174.35
S$17861
  Bottom 0: 169.44,174.35 168.93,174.35
S$17862
  Bottom 0: 168.93,174.35 168.42,174.26
S$17863
  Bottom 0: 168.42,174.26 167.92,174.1
S$17864
  Bottom 0: 167.92,174.1 167.47,173.85
S$17865
  Bottom 0: 167.47,173.85 167.06,173.53
S$17866
  Bottom 0: 167.06,173.53 166.71,173.15
S$17867
  Bottom 0: 166.71,173.15 166.43,172.72
S$17868
  Bottom 0: 166.43,172.72 166.22,172.24
S$17869
  Bottom 0: 166.22,172.24 166.09,171.75
S$17870
  Bottom 0: 166.09,171.75 166.05,171.23
S$17871
  Bottom 0: 166.05,171.23 166.09,170.71
S$17872
  Bottom 0: 166.09,170.71 166.22,170.21
S$17873
  Bottom 0: 166.22,170.21 166.43,169.73
S$17874
  Bottom 0: 166.43,169.73 166.71,169.3
S$17875
  Bottom 0: 166.71,169.3 167.06,168.92
S$17876
  Bottom 0: 167.06,168.92 167.47,168.6
S$17877
  Bottom 0: 167.47,168.6 167.92,168.36
S$17878
  Bottom 0: 167.92,168.36 168.42,168.19
S$17879
  Bottom 0: 168.42,168.19 168.93,168.1
S$17880
  Bottom 0: 321.73,165.74 321.67,165.89
S$17881
  Bottom 0: 321.67,165.89 321.46,166.14
S$17882
  Bottom 0: 321.46,166.14 321.19,166.33
S$17883
  Bottom 0: 321.19,166.33 320.89,166.44
S$17884
  Bottom 0: 320.89,166.44 320.56,166.46
S$17885
  Bottom 0: 320.56,166.46 320.24,166.39
S$17886
  Bottom 0: 320.24,166.39 319.95,166.24
S$17887
  Bottom 0: 319.95,166.24 319.78,166.07
S$17888
  Bottom 0: 319.78,166.07 319.78,169.67
S$17889
  Bottom 0: 319.78,169.67 319.92,169.66
S$17890
  Bottom 0: 319.92,169.66 320.23,169.72
S$17891
  Bottom 0: 320.23,169.72 320.33,169.68
S$17892
  Bottom 0: 320.33,169.68 320.69,169.66
S$17893
  Bottom 0: 320.69,169.66 321.03,169.72
S$17894
  Bottom 0: 321.03,169.72 321.35,169.88
S$17895
  Bottom 0: 321.35,169.88 321.62,170.1
S$17896
  Bottom 0: 321.62,170.1 321.73,170.26
S$17897
  Bottom 0: 321.73,170.26 321.73,165.74
S$17898
  Bottom 0: 223.02,169.27 221.84,170.45
S$17899
  Bottom 0: 221.84,170.45 221.95,170.72
S$17900
  Bottom 0: 221.95,170.72 222,171.07
S$17901
  Bottom 0: 222,171.07 221.95,171.41
S$17902
  Bottom 0: 221.95,171.41 221.82,171.74
S$17903
  Bottom 0: 221.82,171.74 221.62,172.02
S$17904
  Bottom 0: 221.62,172.02 221.35,172.25
S$17905
  Bottom 0: 221.35,172.25 221.03,172.4
S$17906
  Bottom 0: 221.03,172.4 220.68,172.46
S$17907
  Bottom 0: 220.68,172.46 220.34,172.44
S$17908
  Bottom 0: 220.34,172.44 220,172.33
S$17909
  Bottom 0: 220,172.33 219.71,172.15
S$17910
  Bottom 0: 219.71,172.15 219.47,171.89
S$17911
  Bottom 0: 219.47,171.89 219.47,171.92
S$17912
  Bottom 0: 219.47,171.92 219.72,172.16
S$17913
  Bottom 0: 219.72,172.16 219.78,172.23
S$17914
  Bottom 0: 219.78,172.23 219.82,172.3
S$17915
  Bottom 0: 219.82,172.3 219.86,172.38
S$17916
  Bottom 0: 219.86,172.38 219.88,172.47
S$17917
  Bottom 0: 219.88,172.47 219.88,172.56
S$17918
  Bottom 0: 219.88,172.56 219.88,177.43
S$17919
  Bottom 0: 219.88,177.43 219.88,177.52
S$17920
  Bottom 0: 219.88,177.52 219.86,177.61
S$17921
  Bottom 0: 219.86,177.61 219.82,177.69
S$17922
  Bottom 0: 219.82,177.69 219.78,177.76
S$17923
  Bottom 0: 219.78,177.76 219.72,177.83
S$17924
  Bottom 0: 219.72,177.83 219.16,178.39
S$17925
  Bottom 0: 219.16,178.39 219.2,178.69
S$17926
  Bottom 0: 219.2,178.69 219.17,178.9
S$17927
  Bottom 0: 219.17,178.9 225.89,172.18
S$17928
  Bottom 0: 225.89,172.18 225.89,170.94
S$17929
  Bottom 0: 225.89,170.94 225.83,170.92
S$17930
  Bottom 0: 225.83,170.92 225.59,170.73
S$17931
  Bottom 0: 225.59,170.73 225.42,170.48
S$17932
  Bottom 0: 225.42,170.48 225.33,170.19
S$17933
  Bottom 0: 225.33,170.19 225.33,169.88
S$17934
  Bottom 0: 225.33,169.88 225.42,169.6
S$17935
  Bottom 0: 225.42,169.6 225.59,169.35
S$17936
  Bottom 0: 225.59,169.35 225.69,169.27
S$17937
  Bottom 0: 225.69,169.27 223.02,169.27
S$17938
  Bottom 0.635: 283.77,164.68 283.77,150.71
S$17939
  Bottom 0.635: 283.77,150.71 291.35,143.12
S$17940
  Bottom 0.635: 276.35,112.31 276.35,112.88
S$17941
  Bottom 0.635: 284.67,112.66 284.67,105.77
S$17942
  Bottom 0.635: 284.67,105.77 282.99,104.1
S$17943
  Bottom 0.635: 282.99,104.1 282.12,104.1
S$17944
  Bottom 0.635: 282.12,104.1 276.35,109.87
S$17945
  Bottom 0.635: 276.35,109.87 276.35,112.31
S$17946
  Bottom 0.635: 275.08,112.31 276.35,112.31
S$17947
  Bottom 0.635: 275.08,112.31 275.08,111.17
S$17948
  Bottom 0.635: 275.08,112.88 275.08,112.31
S$17949
  Bottom 0.635: 273.81,112.88 273.81,111.17
S$17950
  Bottom 0.635: 273.81,111.17 275.08,111.17
S$17951
  Bottom 0.635: 288.81,127.88 287.28,129.41
S$17952
  Bottom 0.635: 287.28,129.41 285.61,129.41
S$17953
  Bottom 0.635: 285.61,129.41 284.82,128.63
S$17954
  Bottom 0.635: 284.82,128.63 284.82,125.08
S$17955
  Bottom 0.635: 284.82,125.08 286.14,123.76
S$17956
  Bottom 0.635: 286.14,123.76 286.14,114.13
S$17957
  Bottom 0.635: 286.14,114.13 284.67,112.66
S$17958
  Bottom 0.635: 291.35,143.12 291.49,142.98
S$17959
  Bottom 0.635: 291.49,142.98 291.49,130.56
S$17960
  Bottom 0.635: 291.49,130.56 288.81,127.88
S$17961
  Bottom 0.635: 283.77,164.68 285.05,164.68
S$17962
  Bottom 0.635: 283.46,164.68 283.77,164.68
S$17963
  Bottom 0.635: 289.56,178.38 289.56,175.33
S$17964
  Bottom 0.635: 289.56,175.33 287.5,173.27
S$17965
  Bottom 0.635: 285.05,164.68 285.05,170.82
S$17966
  Bottom 0.635: 285.05,170.82 287.5,173.27
S$17967
  Bottom 0.381: 22.73,152.7 22.73,147.85
S$17968
  Bottom 0.381: 22.73,147.85 21.11,146.23
S$17969
  Bottom 0.381: 21.11,146.23 21.11,126.35
S$17970
  Bottom 0.381: 21.11,126.35 19.13,124.37
S$17971
  Bottom 0.381: 19.13,124.37 19.13,120.86
S$17972
  Bottom 0.381: 19.13,120.86 22.96,117.04
S$17973
  Bottom 0.381: 22.96,117.04 22.96,113.92
S$17974
  Bottom 0.381: 11.05,171.07 22.73,159.38
S$17975
  Bottom 0.381: 22.73,159.38 22.73,152.7
S$17976
  Bottom 0.381: 29.99,152.7 22.73,152.7
S$17977
  Bottom 0.381: 230.12,152.02 217.54,152.02
S$17978
  Bottom 0.381: 217.54,152.02 211.21,158.34
S$17979
  Bottom 0.381: 211.21,158.34 204.92,158.34
S$17980
  Bottom 0.381: 204.92,158.34 197.91,165.35
S$17981
  Bottom 0.381: 197.91,165.35 197.91,168.67
S$17982
  Bottom 0.381: 197.91,168.67 195.26,171.31
S$17983
  Bottom 0.381: 195.26,171.31 195.26,174.53
S$17984
  Bottom 0.381: 195.26,174.53 197.73,176.99
S$17985
  Bottom 0.381: 197.73,176.99 197.73,179.83
S$17986
  Bottom 0.381: 197.73,179.83 197.62,179.94
S$17987
  Bottom 0.381: 197.62,179.94 195.35,179.94
S$17988
  Bottom 0.381: 195.35,179.94 186.48,171.07
S$17989
  Bottom 0.381: 186.48,171.07 182.5,171.07
S$17990
  Bottom 0.381: 224.77,100.24 243.64,119.12
S$17991
  Bottom 0.381: 243.64,119.12 243.64,140.04
S$17992
  Bottom 0.381: 243.64,140.04 231.67,152.02
S$17993
  Bottom 0.381: 231.67,152.02 230.12,152.02
S$17994
  Bottom 0.381: 224.77,100.24 223.93,101.08
S$17995
  Bottom 0.381: 223.93,101.08 219.15,101.08
S$17996
  Bottom 0.381: 219.15,101.08 206.31,113.92
S$17997
  Bottom 0.381: 227.74,94.87 227.74,97.27
S$17998
  Bottom 0.381: 227.74,97.27 224.77,100.24
S$17999
  Bottom 0.381: 101.54,132.97 101.54,139.83
S$18000
  Bottom 0.381: 101.54,139.83 94.64,146.72
S$18001
  Bottom 0.381: 94.64,146.72 90,146.72
S$18002
  Bottom 0.381: 90,146.72 87.08,149.65
S$18003
  Bottom 0.381: 206.31,113.92 207.69,115.3
S$18004
  Bottom 0.381: 207.69,115.3 207.69,131.1
S$18005
  Bottom 0.381: 207.69,131.1 200.82,137.97
S$18006
  Bottom 0.381: 30.1,171.07 24.07,171.07
S$18007
  Bottom 0.381: 24.07,171.07 22.18,169.18
S$18008
  Bottom 0.381: 22.18,169.18 22.18,167.72
S$18009
  Bottom 0.381: 22.18,167.72 24.82,165.09
S$18010
  Bottom 0.381: 24.82,165.09 24.82,158.32
S$18011
  Bottom 0.381: 24.82,158.32 29.65,153.49
S$18012
  Bottom 0.381: 29.65,153.49 29.66,153.5
S$18013
  Bottom 0.381: 29.66,153.5 30.32,153.5
S$18014
  Bottom 0.381: 30.32,153.5 30.79,153.03
S$18015
  Bottom 0.381: 30.79,153.03 30.79,152.37
S$18016
  Bottom 0.381: 30.79,152.37 30.79,152.36
S$18017
  Bottom 0.381: 30.79,152.36 30.98,152.16
S$18018
  Bottom 0.381: 30.98,152.16 32.75,152.16
S$18019
  Bottom 0.381: 32.75,152.16 40.87,144.03
S$18020
  Bottom 0.381: 40.87,144.03 40.58,143.75
S$18021
  Bottom 0.381: 40.58,143.75 40.58,138.95
S$18022
  Bottom 0.381: 40.58,138.95 36.52,134.89
S$18023
  Bottom 0.381: 36.52,134.89 36.52,129.7
S$18024
  Bottom 0.381: 36.52,129.7 46.43,119.79
S$18025
  Bottom 0.381: 46.43,119.79 50.17,119.79
S$18026
  Bottom 0.381: 50.17,119.79 53.91,116.05
S$18027
  Bottom 0.381: 53.91,116.05 53.91,113.92
S$18028
  Bottom 0.381: 40.87,144.03 42.96,146.13
S$18029
  Bottom 0.381: 42.96,146.13 72.08,146.13
S$18030
  Bottom 0.381: 72.08,146.13 74.2,148.25
S$18031
  Bottom 0.381: 248.33,126.48 248.33,108.88
S$18032
  Bottom 0.381: 248.33,108.88 245.22,105.77
S$18033
  Bottom 0.381: 245.22,105.77 245.22,101.32
S$18034
  Bottom 0.381: 245.22,101.32 245.89,100.66
S$18035
  Bottom 0.381: 245.89,100.66 248.02,100.66
S$18036
  Bottom 0.381: 248.02,100.66 251.56,97.12
S$18037
  Bottom 0.381: 251.56,97.12 251.56,94.87
S$18038
  Bottom 0.381: 258.25,145.69 248.33,135.78
S$18039
  Bottom 0.381: 248.33,135.78 248.33,126.48
S$18040
  Bottom 0.381: 258.25,145.69 261.56,142.39
S$18041
  Bottom 0.381: 261.56,142.39 279.15,142.39
S$18042
  Bottom 0.381: 279.15,142.39 281.04,144.28
S$18043
  Bottom 0.381: 281.04,144.28 282.08,144.28
S$18044
  Bottom 0.381: 74.2,148.25 74.2,148.49
S$18045
  Bottom 0.381: 74.2,148.49 77.72,152.02
S$18046
  Bottom 0.381: 81.42,135.64 81.42,141.03
S$18047
  Bottom 0.381: 81.42,141.03 74.2,148.25
S$18048
  Bottom 0.381: 258.25,145.69 252.96,150.99
S$18049
  Bottom 0.381: 252.96,150.99 250.2,150.99
S$18050
  Bottom 0.381: 250.2,150.99 249.17,152.02
S$18051
  Bottom 0.381: 249.17,152.02 241.31,152.02
S$18052
  Bottom 0.381: 241.31,152.02 235.61,157.71
S$18053
  Bottom 0.381: 235.61,157.71 219.29,157.71
S$18054
  Bottom 0.381: 219.29,157.71 213.34,163.67
S$18055
  Bottom 0.381: 213.34,163.67 212.35,163.67
S$18056
  Bottom 0.381: 212.35,163.67 208.96,167.06
S$18057
  Bottom 0.381: 208.96,167.06 205.56,167.06
S$18058
  Bottom 0.381: 205.56,167.06 201.55,171.07
S$18059
  Bottom 0.381: 225.36,113.92 225.36,121.51
S$18060
  Bottom 0.381: 225.36,121.51 223.6,123.27
S$18061
  Bottom 0.381: 223.6,123.27 223.6,126.73
S$18062
  Bottom 0.381: 139.64,132.97 140.4,132.97
S$18063
  Bottom 0.381: 140.4,132.97 147.66,140.23
S$18064
  Bottom 0.381: 147.66,140.23 147.66,146.15
S$18065
  Bottom 0.381: 147.66,146.15 150.16,148.65
S$18066
  Bottom 0.381: 150.16,148.65 150.16,151.08
S$18067
  Bottom 0.381: 150.16,151.08 153.31,154.23
S$18068
  Bottom 0.381: 153.31,154.23 153.31,158.8
S$18069
  Bottom 0.381: 85.11,152.02 74.36,162.77
S$18070
  Bottom 0.381: 74.36,162.77 74.36,164.71
S$18071
  Bottom 0.381: 76.88,113.92 76.88,122.66
S$18072
  Bottom 0.381: 76.88,122.66 85.11,130.9
S$18073
  Bottom 0.381: 85.11,130.9 85.11,152.02
S$18074
  Bottom 0.381: 280.99,143.1 261.35,123.46
S$18075
  Bottom 0.381: 261.35,123.46 261.35,114.19
S$18076
  Bottom 0.381: 261.35,114.19 261.08,113.92
S$18077
  Bottom 0.381: 272.99,152.02 252.4,152.02
S$18078
  Bottom 0.381: 252.4,152.02 246.81,157.6
S$18079
  Bottom 0.381: 246.81,157.6 237.29,157.6
S$18080
  Bottom 0.381: 237.29,157.6 226.07,168.82
S$18081
  Bottom 0.381: 226.07,168.82 222.84,168.82
S$18082
  Bottom 0.381: 222.84,168.82 220.6,171.07
S$18083
  Bottom 0.381: 96.77,152.02 85.11,152.02
S$18084
  Bottom 0.381: 281.74,94.85 276.91,94.85
S$18085
  Bottom 0.381: 276.91,94.85 270.51,101.24
S$18086
  Bottom 0.381: 270.51,101.24 270.51,104.48
S$18087
  Bottom 0.381: 270.51,104.48 261.08,113.92
S$18088
  Bottom 0.381: 123.93,147.85 123.93,150.81
S$18089
  Bottom 0.381: 123.93,150.81 108.17,166.58
S$18090
  Bottom 0.381: 108.17,166.58 104.53,166.58
S$18091
  Bottom 0.381: 104.53,166.58 101.91,163.95
S$18092
  Bottom 0.381: 101.91,163.95 97.75,163.95
S$18093
  Bottom 0.381: 97.75,163.95 95.13,166.58
S$18094
  Bottom 0.381: 95.13,166.58 91.74,166.58
S$18095
  Bottom 0.381: 91.74,166.58 87.25,171.07
S$18096
  Bottom 0.381: 113.64,112.75 113.64,120.98
S$18097
  Bottom 0.381: 113.64,120.98 123.93,131.27
S$18098
  Bottom 0.381: 123.93,131.27 123.93,147.85
S$18099
  Bottom 0.381: 123.93,147.85 130.71,147.85
S$18100
  Bottom 0.381: 130.71,147.85 134.87,152.02
S$18101
  Bottom 0.381: 286.9,146.22 275.49,157.62
S$18102
  Bottom 0.381: 275.49,157.62 267.49,157.62
S$18103
  Bottom 0.381: 267.49,157.62 266.65,158.46
S$18104
  Bottom 0.381: 266.65,158.46 266.65,169.49
S$18105
  Bottom 0.381: 266.65,169.49 268.22,171.07
S$18106
  Bottom 0.381: 177.74,132.97 177.74,140.52
S$18107
  Bottom 0.381: 177.74,140.52 172.4,145.86
S$18108
  Bottom 0.381: 111.06,113.92 111.06,100.09
S$18109
  Bottom 0.381: 111.06,100.09 104.78,93.81
S$18110
  Bottom 0.381: 301.51,143.12 292.42,134.03
S$18111
  Bottom 0.381: 292.42,134.03 292.42,131.45
S$18112
  Bottom 0.381: 320.21,95.23 319.83,94.85
S$18113
  Bottom 0.381: 320.6,152 321.96,150.63
S$18114
  Bottom 0.381: 321.96,150.63 321.96,96.98
S$18115
  Bottom 0.381: 321.96,96.98 320.21,95.23
S$18116
  Bottom 0.381: 320.59,94.85 320.21,95.23
S$18117
  Bottom 0.381: 203.93,94.87 206.13,92.67
S$18118
  Bottom 0.381: 206.13,92.67 215.48,92.67
S$18119
  Bottom 0.381: 215.48,92.67 216.73,93.92
S$18120
  Bottom 0.381: 216.73,93.92 224.02,93.92
S$18121
  Bottom 0.381: 224.02,93.92 224.66,93.28
S$18122
  Bottom 0.381: 224.66,93.28 228.3,93.28
S$18123
  Bottom 0.381: 228.3,93.28 246.46,111.44
S$18124
  Bottom 0.381: 246.46,111.44 246.46,139.23
S$18125
  Bottom 0.381: 212.14,153.08 207.5,157.72
S$18126
  Bottom 0.381: 207.5,157.72 204.75,157.72
S$18127
  Bottom 0.381: 204.75,157.72 199.9,162.57
S$18128
  Bottom 0.381: 199.9,162.57 194.4,162.57
S$18129
  Bottom 0.381: 194.4,162.57 190.35,166.61
S$18130
  Bottom 0.381: 190.35,166.61 180.77,166.61
S$18131
  Bottom 0.381: 180.77,166.61 178.12,163.95
S$18132
  Bottom 0.381: 178.12,163.95 174.33,163.95
S$18133
  Bottom 0.381: 174.33,163.95 171.52,166.77
S$18134
  Bottom 0.381: 171.52,166.77 167.75,166.77
S$18135
  Bottom 0.381: 167.75,166.77 163.45,171.07
S$18136
  Bottom 0.381: 212.14,153.08 223.37,141.85
S$18137
  Bottom 0.381: 223.37,141.85 240.65,141.85
S$18138
  Bottom 0.381: 240.65,141.85 242.84,139.65
S$18139
  Bottom 0.381: 211.07,152.02 212.14,153.08
S$18140
  Bottom 0.381: 82.49,132.97 83.84,134.32
S$18141
  Bottom 0.381: 83.84,134.32 83.84,148.03
S$18142
  Bottom 0.381: 83.84,148.03 74.91,156.97
S$18143
  Bottom 0.381: 74.91,156.97 44.57,156.97
S$18144
  Bottom 0.381: 44.57,156.97 39.62,152.02
S$18145
  Bottom 0.381: 203.93,94.87 203.93,101.8
S$18146
  Bottom 0.381: 203.93,101.8 196.43,109.3
S$18147
  Bottom 0.381: 196.43,109.3 191.88,109.3
S$18148
  Bottom 0.381: 191.88,109.3 187.26,113.92
S$18149
  Bottom 0.381: 265.84,132.97 273.01,140.13
S$18150
  Bottom 0.381: 115.82,152.02 115.82,154.27
S$18151
  Bottom 0.381: 115.82,154.27 112.38,157.71
S$18152
  Bottom 0.381: 112.38,157.71 110.3,157.71
S$18153
  Bottom 0.381: 110.3,157.71 105.32,162.69
S$18154
  Bottom 0.381: 105.32,162.69 105.32,162.88
S$18155
  Bottom 0.381: 104.31,117.46 107.24,120.39
S$18156
  Bottom 0.381: 107.24,120.39 107.24,122.96
S$18157
  Bottom 0.381: 107.24,122.96 110.5,126.23
S$18158
  Bottom 0.381: 110.5,126.23 112.31,126.23
S$18159
  Bottom 0.381: 112.31,126.23 116.65,130.57
S$18160
  Bottom 0.381: 116.65,130.57 116.65,131.86
S$18161
  Bottom 0.381: 116.65,131.86 121.96,137.16
S$18162
  Bottom 0.381: 121.96,137.16 121.96,145.88
S$18163
  Bottom 0.381: 121.96,145.88 115.82,152.02
S$18164
  Bottom 0.381: 283.54,141.81 283.63,141.81
S$18165
  Bottom 0.381: 283.54,141.81 283.54,146.75
S$18166
  Bottom 0.381: 283.54,146.75 273.22,157.06
S$18167
  Bottom 0.381: 273.22,157.06 265.04,157.06
S$18168
  Bottom 0.381: 265.04,157.06 264.7,157.41
S$18169
  Bottom 0.381: 264.7,157.41 259.2,157.41
S$18170
  Bottom 0.381: 259.2,157.41 258.72,156.93
S$18171
  Bottom 0.381: 258.72,156.93 255.22,156.93
S$18172
  Bottom 0.381: 255.22,156.93 250.9,161.25
S$18173
  Bottom 0.381: 250.9,161.25 248.76,161.25
S$18174
  Bottom 0.381: 248.76,161.25 239.65,170.37
S$18175
  Bottom 0.381: 239.65,170.37 239.65,171.07
S$18176
  Bottom 0.381: 271.21,127.61 271.21,129.48
S$18177
  Bottom 0.381: 271.21,129.48 283.54,141.81
S$18178
  Bottom 0.381: 158.69,132.97 158.69,141.39
S$18179
  Bottom 0.381: 158.69,141.39 155.05,145.02
S$18180
  Bottom 0.381: 300.27,95.37 299.82,94.92
S$18181
  Bottom 0.381: 299.82,94.92 289.95,94.92
S$18182
  Bottom 0.381: 289.95,94.92 284.84,100.03
S$18183
  Bottom 0.381: 284.84,100.03 276.78,100.03
S$18184
  Bottom 0.381: 276.78,100.03 271.21,105.6
S$18185
  Bottom 0.381: 271.21,105.6 271.21,127.61
S$18186
  Bottom 0.381: 271.21,127.61 267.88,127.61
S$18187
  Bottom 0.381: 300.27,95.37 300.79,94.85
S$18188
  Bottom 0.381: 300.79,113.9 300.27,113.38
S$18189
  Bottom 0.381: 300.27,113.38 300.27,95.37
S$18190
  Bottom 0.381: 300.78,152 300.78,144.94
S$18191
  Bottom 0.381: 300.78,144.94 298.97,143.12
S$18192
  Bottom 0.381: 153.92,152.02 154.24,152.33
S$18193
  Bottom 0.381: 154.24,152.33 154.24,159
S$18194
  Bottom 0.381: 154.24,159 149.01,164.24
S$18195
  Bottom 0.381: 149.01,164.24 145.41,164.24
S$18196
  Bottom 0.381: 145.41,164.24 145.01,163.83
S$18197
  Bottom 0.381: 145.01,163.83 135.97,163.83
S$18198
  Bottom 0.381: 135.97,163.83 133.23,166.58
S$18199
  Bottom 0.381: 133.23,166.58 122.76,166.58
S$18200
  Bottom 0.381: 122.76,166.58 120.14,163.95
S$18201
  Bottom 0.381: 120.14,163.95 116.8,163.95
S$18202
  Bottom 0.381: 116.8,163.95 113.62,167.14
S$18203
  Bottom 0.381: 113.62,167.14 110.23,167.14
S$18204
  Bottom 0.381: 110.23,167.14 106.3,171.07
S$18205
  Bottom 0.381: 122.18,109.94 115.59,116.54
S$18206
  Bottom 0.381: 115.59,116.54 115.59,120.91
S$18207
  Bottom 0.381: 115.59,120.91 123.48,128.81
S$18208
  Bottom 0.381: 123.48,128.81 137.68,128.81
S$18209
  Bottom 0.381: 137.68,128.81 149,140.13
S$18210
  Bottom 0.381: 149,140.13 149,146.3
S$18211
  Bottom 0.381: 149,146.3 153.92,151.22
S$18212
  Bottom 0.381: 153.92,151.22 153.92,152.02
S$18213
  Bottom 0.381: 37.24,94.87 25.73,94.87
S$18214
  Bottom 0.381: 25.73,94.87 22.26,91.4
S$18215
  Bottom 0.381: 22.26,91.4 16.91,91.4
S$18216
  Bottom 0.381: 16.91,91.4 16.17,92.14
S$18217
  Bottom 0.381: 16.17,92.14 16.17,94.28
S$18218
  Bottom 0.381: 16.17,94.28 9.61,100.83
S$18219
  Bottom 0.381: 9.61,100.83 9.61,124.38
S$18220
  Bottom 0.381: 9.61,124.38 18.19,132.97
S$18221
  Bottom 0.381: 122.18,109.94 105.25,93
S$18222
  Bottom 0.381: 105.25,93 56.8,93
S$18223
  Bottom 0.381: 56.8,93 54.28,95.52
S$18224
  Bottom 0.381: 54.28,95.52 37.9,95.52
S$18225
  Bottom 0.381: 37.9,95.52 37.24,94.87
S$18226
  Bottom 0.381: 122.18,109.94 122.4,109.73
S$18227
  Bottom 0.381: 122.4,109.73 125.93,109.73
S$18228
  Bottom 0.381: 125.93,109.73 130.11,113.92
S$18229
  Bottom 0.381: 196.79,132.97 196.79,135.09
S$18230
  Bottom 0.381: 196.79,135.09 193.22,138.66
S$18231
  Bottom 0.381: 193.22,138.66 191.11,138.66
S$18232
  Bottom 0.381: 191.11,138.66 188.78,140.99
S$18233
  Bottom 0.381: 188.78,140.99 188.78,141.21
S$18234
  Bottom 0.381: 301.55,171.05 304.05,168.54
S$18235
  Bottom 0.381: 304.05,168.54 304.05,143.12
S$18236
  Bottom 0.381: 158.12,152.26 157.66,151.79
S$18237
  Bottom 0.381: 157.66,151.79 157.07,151.79
S$18238
  Bottom 0.381: 157.07,151.79 149.77,144.5
S$18239
  Bottom 0.381: 149.77,144.5 149.77,138.05
S$18240
  Bottom 0.381: 149.77,138.05 144.18,132.46
S$18241
  Bottom 0.381: 144.18,132.46 144.18,128.37
S$18242
  Bottom 0.381: 144.18,128.37 145.63,126.91
S$18243
  Bottom 0.381: 144.4,171.07 144.4,170.43
S$18244
  Bottom 0.381: 144.4,170.43 158.12,156.7
S$18245
  Bottom 0.381: 158.12,156.7 158.12,152.26
S$18246
  Bottom 0.381: 158.12,152.26 158.28,152.11
S$18247
  Bottom 0.381: 158.28,152.11 170.46,152.11
S$18248
  Bottom 0.381: 170.46,152.11 171.91,153.56
S$18249
  Bottom 0.381: 171.91,153.56 175.58,153.56
S$18250
  Bottom 0.381: 175.58,153.56 176.98,152.16
S$18251
  Bottom 0.381: 176.98,152.16 192.02,152.16
S$18252
  Bottom 0.381: 63.44,132.97 54.75,132.97
S$18253
  Bottom 0.381: 54.75,132.97 46.14,141.57
S$18254
  Bottom 0.381: 46.14,141.57 46.14,144.31
S$18255
  Bottom 0.381: 147.53,109.75 147.53,115.12
S$18256
  Bottom 0.381: 147.53,115.12 148,115.58
S$18257
  Bottom 0.381: 148,115.58 148,123.2
S$18258
  Bottom 0.381: 148,123.2 147.31,123.89
S$18259
  Bottom 0.381: 147.31,123.89 147.31,126.33
S$18260
  Bottom 0.381: 147.31,126.33 147.88,126.9
S$18261
  Bottom 0.381: 192.02,152.16 192.02,152.02
S$18263
  Bottom 0.381: 234.89,132.97 224.84,132.97
S$18264
  Bottom 0.381: 224.84,132.97 199.2,158.6
S$18265
  Bottom 0.381: 199.2,158.6 199.2,158.84
S$18266
  Bottom 0.381: 199.2,158.84 198.29,159.74
S$18267
  Bottom 0.381: 198.29,159.74 197.07,159.74
S$18268
  Bottom 0.381: 197.07,159.74 192.02,154.69
S$18269
  Bottom 0.381: 192.02,154.69 192.02,152.16
S$18270
  Bottom 0.381: 147.53,109.75 147.38,109.75
S$18271
  Bottom 0.381: 147.38,109.75 132.5,94.87
S$18272
  Bottom 0.381: 168.21,113.92 164.04,109.75
S$18273
  Bottom 0.381: 164.04,109.75 147.53,109.75
S$18274
  Bottom 0.381: 157.32,152.6 157.32,156.71
S$18275
  Bottom 0.381: 157.32,156.71 147.46,166.58
S$18276
  Bottom 0.381: 147.46,166.58 142.49,166.58
S$18277
  Bottom 0.381: 142.49,166.58 137.79,171.27
S$18278
  Bottom 0.381: 172.97,152.02 168.79,147.84
S$18279
  Bottom 0.381: 168.79,147.84 155.93,147.84
S$18280
  Bottom 0.381: 155.93,147.84 154.16,146.07
S$18281
  Bottom 0.381: 154.16,146.07 154.16,144.78
S$18282
  Bottom 0.381: 154.16,144.78 157.54,141.4
S$18283
  Bottom 0.381: 157.54,141.4 157.54,134.61
S$18284
  Bottom 0.381: 157.54,134.61 157.11,134.19
S$18285
  Bottom 0.381: 157.11,134.19 157.11,133.06
S$18286
  Bottom 0.381: 157.11,133.06 151.99,127.94
S$18287
  Bottom 0.381: 151.99,127.94 150.48,127.94
S$18288
  Bottom 0.381: 150.48,127.94 147.87,125.33
S$18289
  Bottom 0.381: 147.87,125.33 147.87,124.17
S$18290
  Bottom 0.381: 147.87,124.17 149.16,122.88
S$18291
